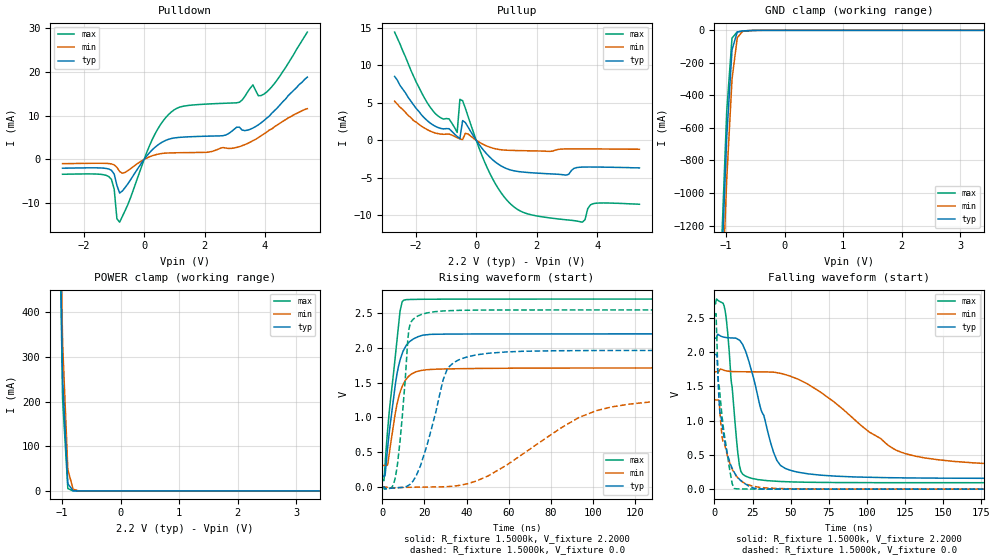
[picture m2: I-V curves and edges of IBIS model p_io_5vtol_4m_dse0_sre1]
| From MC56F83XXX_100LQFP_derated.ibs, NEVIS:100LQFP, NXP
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[Model] p_io_5vtol_4m_dse0_sre1
|   Model p_io_5vtol_4m_dse0_sre1
| Library cells for typ/min/max conditions are connected as defined below:
|  pad - External Pad
|  ipp_do - Core Input
|  ipp_obe - Output Buffer Enable
|  esd_boost - vdd_s_3v
|  esd_bus - vdd_s_3v
|  ipp_ame - vss_s_lv
|  ipp_dse - vss_s_lv
|  ipp_ina40a_5vtol - NC
|  ipp_ina40b_5vtol - NC
|  ipp_ina_5vtol - NC
|  ipp_ina_mux_3v - NC
|  ipp_ind - NC
|  ipp_ind_3v - NC
|  ipp_pue - vss_s_lv
|  ipp_sre - vdd_s_lv
|  tie_3v - vdd_s_3v
|  tie_hi - vdd_s_lv
|  vbuf_3v - vdd_s_3v
|  vdd_bulk_lv - vdd_s_lv
|  vdd_s_3v - vdd_s_3v
|  vdd_s_lv - vdd_s_lv
|  vss_bulk - vss_s_3v
|  vss_s_3v - vss_s_3v
|  vss_s_lv - vss_s_lv
| All other pins connected to ground
Model_type I/O
Polarity   Non-Inverting
Enable   Active-High
Vinl =   0.7700V
Vinh =   1.5400V
Vmeas =  1.1000V
Cref =   25.0000pF
Rref =   1.0000k
Vref =   0.0V
C_comp   2.5897pF   2.5141pF   2.6932pF
[Temperature Range]   25.0000   0.1250k   -40.0000
[Voltage Range]   2.2000V   1.7100V   2.7000V
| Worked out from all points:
|   slope of the pulldown table from 0 to 0.33 V, typ, clamps not added: 128 ohm
|   slope of the pullup table from 0 to 0.33 V, typ, clamps not added: 190 ohm
|   GND clamp passes 1 mA (typ) near -0.56 V on its own axis
|   POWER clamp passes 1 mA (typ) near -0.81 V on its own axis
|   rising waveform, R_fixture 1.5000k, V_fixture 2.2000: 20-80 % time 5.65ns typ, 5.46ns min, 5.16ns max; typ from 0.156 V to 2.2 V
|   rising waveform, R_fixture 1.5000k, V_fixture 0.0: 20-80 % time 10.2ns typ, 40.8ns min, 4.04ns max; typ from 0 V to 1.96 V
|   falling waveform, R_fixture 1.5000k, V_fixture 2.2000: 20-80 % time 14.9ns typ, 48.1ns min, 5.86ns max; typ from 2.2 V to 0.157 V
|   falling waveform, R_fixture 1.5000k, V_fixture 0.0: 20-80 % time 7.69ns typ, 8.52ns min, 6.7ns max; typ from 1.96 V to 0 V
[Pulldown]
|Voltage   I(typ)   I(min)   I(max)
-2.7V     -2mA       -960uA     -3.39mA
-1.17V    -2.19mA    -943uA     -3.913mA
-990mV    -3.359mA   -1.244mA   -6.804mA
-900mV    -5.941mA   -1.821mA   -13.58mA
-810mV    -7.677mA   -2.75mA    -14.34mA
270mV     2.201mA    843.6uA    4.568mA
810mV     4.605mA    1.475mA    10.28mA
3.15V     7.385mA    2.91mA     13.07mA
3.6V      7.17mA     4.3mA      17.03mA
3.78V     7.91mA     5mA        14.56mA
3.96V     8.86mA     5.8mA      14.91mA
5.4V      18.8mA     11.6mA     29.1mA
[Pullup]
|Voltage   I(typ)   I(min)   I(max)
-2.7V     8.5mA      5.2mA      14.4mA
-1.35V    1.85mA     960uA      3.54mA
-630mV    503.1uA    337.6uA    1.039mA
-540mV    232uA      184.5uA    5.441mA
-450mV    2.62mA     76.25uA    5.267mA
-270mV    1.759mA    833.9uA    3.181mA
450mV     -2.247mA   -924uA     -4.401mA
1.35V     -4.138mA   -1.371mA   -9.168mA
2.97V     -4.634mA   -1.154mA   -10.59mA
3.51V     -3.575mA   -1.148mA   -10.91mA
3.87V     -3.565mA   -1.16mA    -8.446mA
5.4V      -3.68mA    -1.2mA     -8.52mA
[GND_clamp]
|Voltage   I(typ)   I(min)   I(max)
-2.7V     -20.35A    -20.38A    -20.37A
-1.08V    -1.486A    -1.737A    -1.339A
-990mV    -654.8mA   -915.7mA   -496.6mA
-900mV    -120.3mA   -300.6mA   -47.98mA
-810mV    -10.43mA   -45.61mA   -9.206mA
-720mV    -3.577mA   -6.172mA   -6.342mA
-540mV    -682.6uA   -563.7uA   -1.265mA
5.4V      0A         0A         0A
[POWER_clamp]
|Voltage   I(typ)   I(min)   I(max)
-2.7V     20.23A     19.96A     20.45A
-1.08V    950.5mA    990.2mA    948mA
-990mV    252.7mA    333.8mA    206.6mA
-900mV    16.05mA    47.59mA    5.278mA
-810mV    508.3uA    3.841mA    61.17uA
-720mV    15.33uA    281.3uA    694.4nA
-630mV    461.8nA    20.43uA    7.955nA
5.4V      0A         0A         0A
[Ramp]
| variable   typ   min   max
dV/dt_r  0.1311/23.4035n   41.8663m/52.4404n   0.3060/12.8070n
dV/dt_f  0.1582/45.1695n   44.5644m/78.6097n   0.3795/25.2219n
R_load = 50.0000
[Rising Waveform]
R_fixture= 1.5000k
V_fixture= 2.2000
V_fixture_min= 1.7100
V_fixture_max= 2.7000
|time   V(typ)   V(min)   V(max)
0s        156.3mV    309.1mV    94.08mV
815.6ps   157.1mV    309.1mV    105.6mV
1.298ns   167.8mV    309.1mV    331.9mV
2.604ns   593.5mV    333.2mV    856.3mV
6.029ns   1.445V     1.038V     1.844V
7.679ns   1.734V     1.282V     2.341V
8.414ns   1.822V     1.361V     2.529V
10.15ns   1.968V     1.489V     2.684V
22.89ns   2.193V     1.688V     2.698V
250ns     2.2V       1.71V      2.7V
[Rising Waveform]
R_fixture= 1.5000k
V_fixture= 0.0
V_fixture_min= 0.0
V_fixture_max= 0.0
|time   V(typ)   V(min)   V(max)
0s        2.604nV    511.6nV    74.27pV
5.747ns   -13.5mV    -12mV      81.86mV
8.324ns   -9.099mV   -8.182mV   632.2mV
12.6ns    26.88mV    -4.742mV   2.258V
18.59ns   350.7mV    -2.482mV   2.479V
30.52ns   1.672V     3.915mV    2.532V
40.3ns    1.869V     45.21mV    2.54V
93.45ns   1.96V      998.7mV    2.543V
108.8ns   1.961V     1.149V     2.544V
250ns     1.962V     1.298V     2.544V
[Falling Waveform]
R_fixture= 1.5000k
V_fixture= 2.2000
V_fixture_min= 1.7100
V_fixture_max= 2.7000
|time   V(typ)   V(min)   V(max)
0s        2.2V       1.71V      2.7V
6.944ns   2.212V     1.727V     2.608V
8.52ns    2.207V     1.72V      2.32V
15.27ns   2.186V     1.711V     541.7mV
17.35ns   2.146V     1.711V     258.9mV
20.57ns   2.003V     1.71V      188.7mV
38.71ns   541.7mV    1.704V     117.1mV
48.84ns   281.9mV    1.654V     106.5mV
126.3ns   163.9mV    510.7mV    94.31mV
250ns     156.6mV    328.6mV    94.08mV
[Falling Waveform]
R_fixture= 1.5000k
V_fixture= 0.0
V_fixture_min= 0.0
V_fixture_max= 0.0
|time   V(typ)   V(min)   V(max)
0s        1.962V     1.299V     2.544V
1.008ns   1.962V     1.299V     2.55V
1.612ns   1.955V     1.299V     2.128V
2.553ns   1.492V     1.3V       1.576V
3.481ns   1.132V     1.164V     1.404V
4.807ns   982mV      800.2mV    1.092V
8.792ns   484.8mV    465.6mV    459.7mV
12.95ns   246mV      239.2mV    12.26mV
30.99ns   2.45mV     24.33mV    945.8uV
250ns     336.6nV    50.98uV    -9.618nV
